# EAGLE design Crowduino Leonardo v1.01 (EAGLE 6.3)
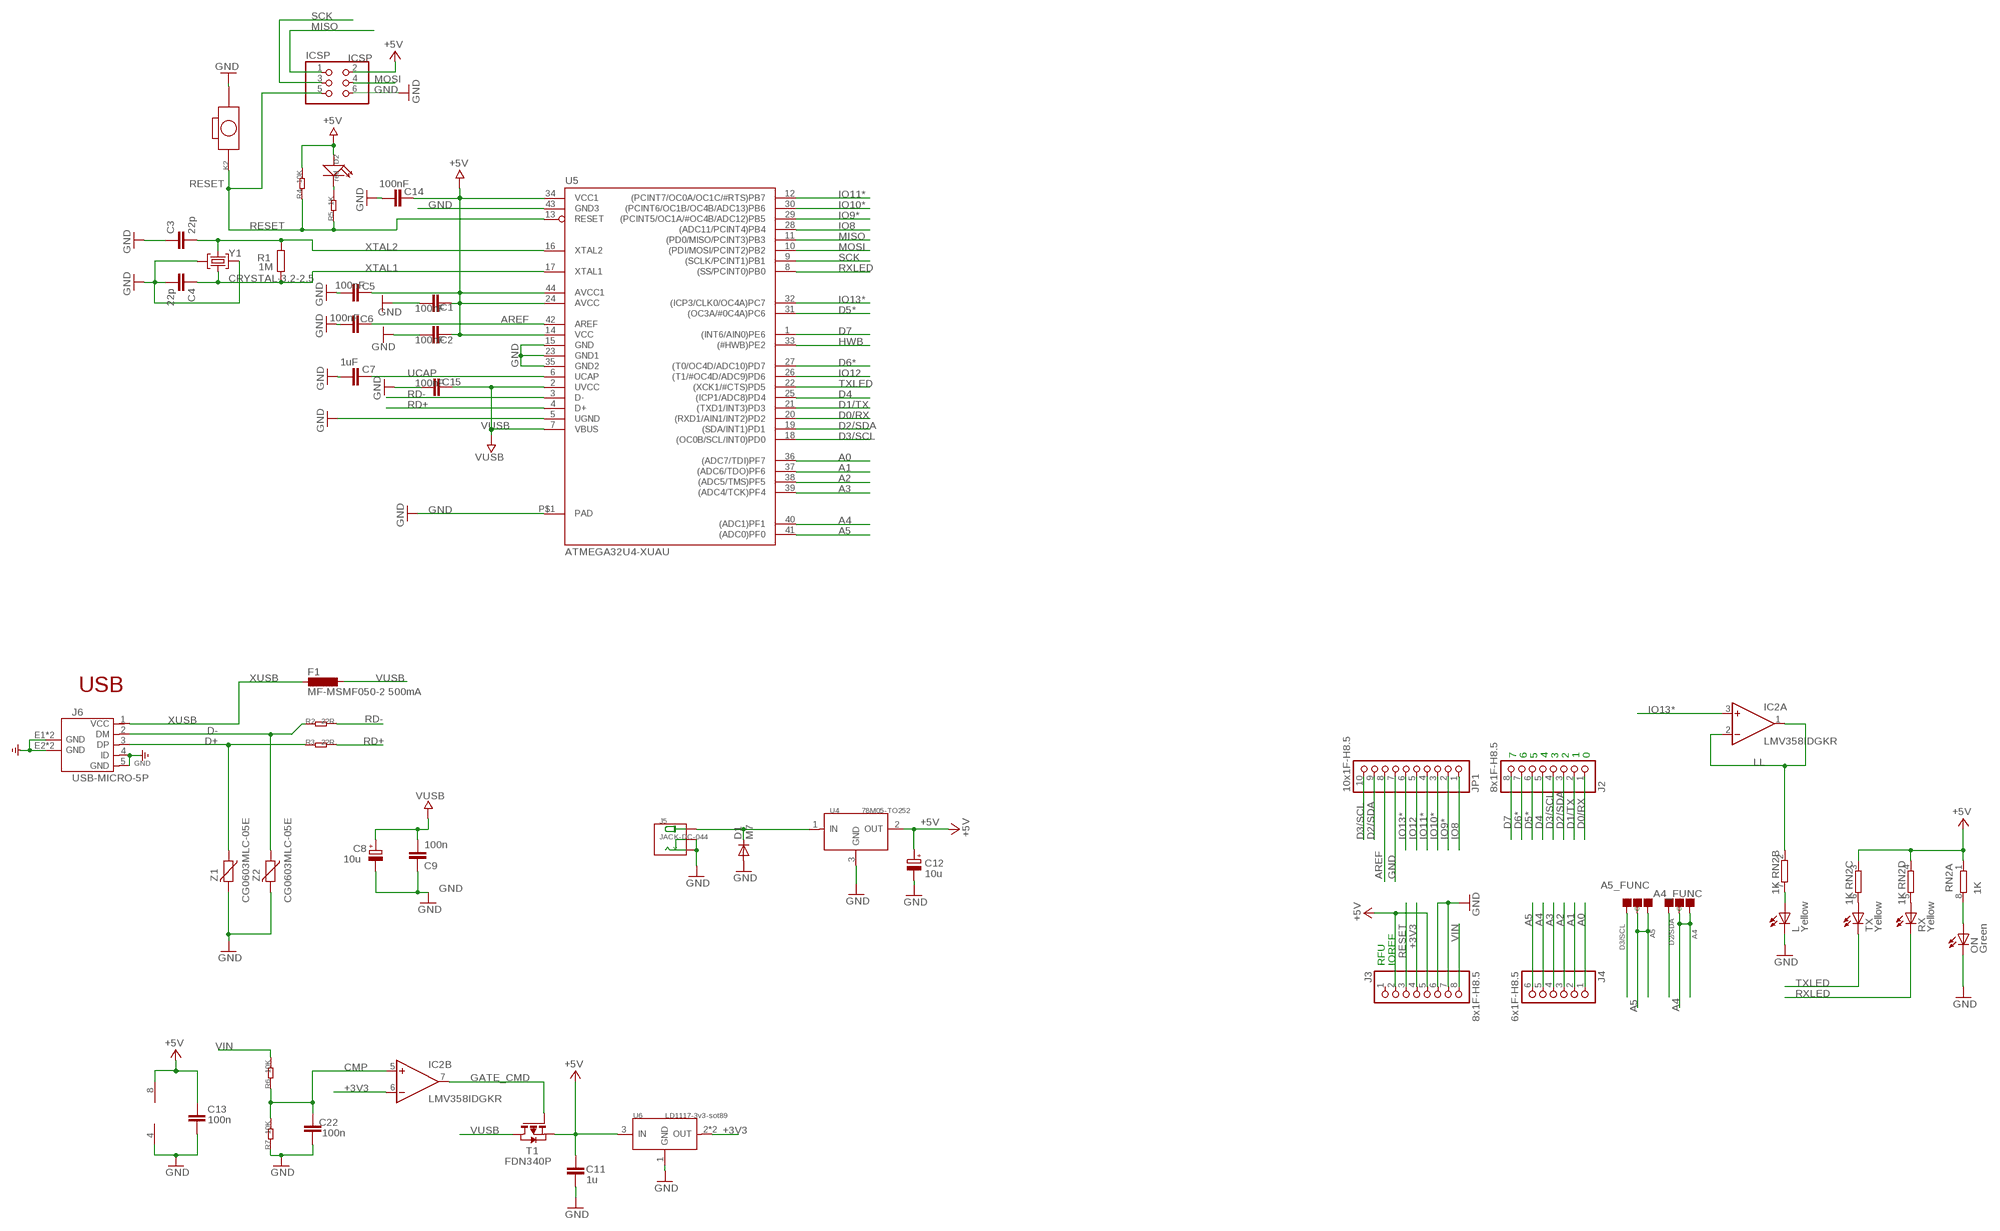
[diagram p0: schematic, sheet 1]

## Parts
A4_FUNC  DNP  PAD-JUMPER-3P-40*40  [3P-SMD-4.1X1.5]
A5_FUNC  DNP  PAD-JUMPER-3P-40*40  [3P-SMD-4.1X1.5]
C1  100nF  C-EUC0603  [C0603-ROUND]
C2  100nF  C-EUC0603  [C0603-ROUND]
C3  22p  C-EUC0603  [C0603-ROUND]
C4  22p  C-EUC0603  [C0603-ROUND]
C5  100nF  C-EUC0603  [C0603-ROUND]
C6  100nF  C-EUC0603  [C0603-ROUND]
C7  1uF  C-EUC0603  [C0603-ROUND]
C8  10u  CPOL-EUSMCB  [SMC_B]
C9  100n  C-EUC0603  [C0603-ROUND]
C11  1u  C-EUC0603  [C0603-ROUND]
C12  10u  CPOL-EUSMCB  [SMC_B]
C13  100n  C-EUC0603  [C0603-ROUND]
C14  100nF  C-EUC0603  [C0603-ROUND]
C15  100nF  C-EUC0603  [C0603-ROUND]
C22  100n  C-EUC0603  [C0603-ROUND]
D1  M7  DIODE-SMB  [SMB]
D2  red  LED'0603'  [LED-0603]
F1  MF-MSMF050-2 500mA  L-EUL1812  [L1812]
IC2  LMV358IDGKR  LMV358MMX  [MSOP08]
ICSP  ICSP  PINHD-2X3  [2X03]
J2  8x1F-H8.5  PINHD-1X8  [1X08]
J3  8x1F-H8.5  PINHD-1X8  [1X08]
J4  6x1F-H8.5  PINHD-1X6  [1X06]
J5  JACK-DC-044  [DC-404]
J6  USB-MICRO-5P  [MICRO-USB-5P]
JP1  10x1F-H8.5  PINHD-1X10  [1X10]
K2  BOTTON-2P-90D  [2P-7.62X3.56-90D]
L  Yellow  LEDCHIPLED_0805  [CHIPLED_0805]
ON  Green  LEDCHIPLED_0805  [CHIPLED_0805]
R1  1M  R-EU_R0603  [R0603-ROUND]
R2  22R  R-0603  [R0603]
R3  22R  R-0603  [R0603]
R4  10K  R-0603  [R0603]
R5  1K  R-0603  [R0603]
R6  10K  R-0603  [R0603]
R7  10K  R-0603  [R0603]
RN2  1K  4R-NCAY16  [CAY16]
RX  Yellow  LEDCHIPLED_0805  [CHIPLED_0805]
T1  FDN340P  PMOSSOT23  [SOT-23]
TX  Yellow  LEDCHIPLED_0805  [CHIPLED_0805]
U4  78M05-TO252  [TO252]
U5  ATMEGA32U4-XUAU  [TQFP44-PAD]
U6  LD1117-3v3-sot89  LD1117'SOT89'  [SOT89]
Y1  CRYSTAL-3.2-2.5  [CRYSTAL-3.2-2.5]
Z1  CG0603MLC-05E  VARISTORCN0603  [CT/CN0603]
Z2  CG0603MLC-05E  VARISTORCN0603  [CT/CN0603]

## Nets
+3V3: IC2.6(B:-IN) J3.4 U6.2(OUT) U6.4(OUT)
+5V [usbvcc]: C1.1 C2.1 C5.1 C11.2 C12.+ C13.1 C14.1 D2.+ IC2.8(P:V+) ICSP.2 J3.2 J3.5 R4.2 RN2.1 RN2.3 RN2.4 T1.2(S) U4.2(OUT) U5.14(VCC) U5.24(AVCC) U5.34(VCC1) U5.44(AVCC1) U6.3(IN)
A0: J4.1 U5.36((ADC7/TDI)PF7)
A1: J4.2 U5.37((ADC6/TDO)PF6)
A2: J4.3 U5.38((ADC5/TMS)PF5)
A3: J4.4 U5.39((ADC4/TCK)PF4)
A4: A4_FUNC.00(L) A4_FUNC.MM(C) J4.5 U5.40((ADC1)PF1)
A5: A5_FUNC.00(L) A5_FUNC.MM(C) J4.6 U5.41((ADC0)PF0)
AREF [aref]: C6.2 JP1.8 U5.42(AREF)
CMP: C22.2 IC2.5(B:+IN) R6.1 R7.2
D0/RX: J2.1 U5.20((RXD1/AIN1/INT2)PD2)
D1/TX: J2.2 U5.21((TXD1/INT3)PD3)
D2/SDA: A4_FUNC.11(R) J2.3 JP1.9 U5.19((SDA/INT1)PD1)
D3/SCL: A5_FUNC.11(R) J2.4 JP1.10 U5.18((OC0B/SCL/INT0)PD0)
D4: J2.5 U5.25((ICP1/ADC8)PD4)
D5*: J2.6 U5.31((OC3A/#0C4A)PC6)
D6*: J2.7 U5.27((T0/OC4D/ADC10)PD7)
D7: J2.8 U5.1((INT6/AIN0)PE6)
D+: J6.3(DP) R3.1 Z1.1
D-: J6.2(DM) R2.1 Z2.1
GATE_CMD: IC2.7(B:OUT) T1.3(G)
GND [gnd]: C1.2 C2.2 C3.1 C4.2 C5.2 C6.1 C7.2 C8.- C9.1 C11.1 C12.- C13.2 C14.2 C15.2 C22.1 D1.A IC2.4(P:V-) ICSP.6 J3.6 J3.7 J5.- J5.CDN J6.4(ID) J6.5(GND) J6.E1(GND) J6.E2(GND) J6.P1(GND) J6.P2(GND) JP1.7 K2.P$2 L.C ON.C R7.1 U4.3(GND) U5.5(UGND) U5.15(GND) U5.23(GND1) U5.35(GND2) U5.43(GND3) U5.P$1(PAD) U6.1(GND) Y1.2(GND) Y1.4(GND) Z1.2 Z2.2
HWB: U5.33((#HWB)PE2)
IO8: JP1.1 U5.28((ADC11/PCINT4)PB4)
IO9*: JP1.2 U5.29((PCINT5/OC1A/#OC4B/ADC12)PB5)
IO10*: JP1.3 U5.30((PCINT6/OC1B/OC4B/ADC13)PB6)
IO11*: JP1.4 U5.12((PCINT7/OC0A/OC1C/#RTS)PB7)
IO12: JP1.5 U5.26((T1/#OC4D/ADC9)PD6)
IO13*: IC2.3(A:+IN) JP1.6 U5.32((ICP3/CLK0/OC4A)PC7)
LL: IC2.1(A:OUT) IC2.2(A:-IN) RN2.2
MISO: ICSP.1 U5.11((PD0/MISO/PCINT3)PB3)
MOSI: ICSP.4 U5.10((PDI/MOSI/PCINT2)PB2)
N$1: D2.- R5.2
N$2: L.A RN2.7
N$3: ON.A RN2.8
N$6: RN2.6 TX.A
N$8: RN2.5 RX.A
RD+: R3.2 U5.4(D+)
RD-: R2.2 U5.3(D-)
RESET: ICSP.5 J3.3 K2.P$1 R4.1 R5.1 U5.13(RESET)
RXLED: RX.C U5.8((SS/PCINT0)PB0)
SCK: ICSP.3 U5.9((SCLK/PCINT1)PB1)
TXLED: TX.C U5.22((XCK1/#CTS)PD5)
UCAP: C7.1 U5.6(UCAP)
VIN [none1]: D1.C J3.8 J5.+ R6.2 U4.1(IN)
VUSB: C8.+ C9.2 C15.1 F1.1 T1.1(D) U5.2(UVCC) U5.7(VBUS)
XTAL1: C4.1 R1.1 U5.17(XTAL1) Y1.1(C1)
XTAL2: C3.2 R1.2 U5.16(XTAL2) Y1.3(C2)
XUSB [usbvcc]: F1.2 J6.1(VCC)
Unconnected: J3.1

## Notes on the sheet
- USB
- 7 | 6 | 5 | 4 | 3 | 2 | 1 | 0
- RFU | IOREF

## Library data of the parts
A4_FUNC A5_FUNC = Discrete:PAD-JUMPER-3P; PARTNO: DNP
C1-C7 C9 C11 C13-C15 C22 = SmartPrj:C-EU: CAPACITOR, European symbol
C8 C12 = rcl:CPOL-EU: POLARIZED CAPACITOR, European symbol
D1 = diode:DIODE-: DIODE
D2 = Discrete:LED*
F1 = rcl:L-EU: INDUCTOR, European symbol
IC2 = linear:LMV358?*: Dual General Purpose, Low Voltage, Rail-to-Rail Output Operational Amplifiers Source: http://www.national.com/mpf/LM/LMV321.html http://www.national.com/dt/lmv_qual.pdf
ICSP = SmartPrj:PINHD-2X3: PIN HEADER
J2 J3 = SmartPrj:PINHD-1X8: PIN HEADER
J4 = SmartPrj:PINHD-1X6: PIN HEADER
J5 = Connector:JACK-DC-044
J6 = Connector:USB-MICRO-5P
JP1 = SmartPrj:PINHD-1X10: PIN HEADER
K2 = Discrete:BOTTON-2P
L ON RX TX = led:LED: LED
R1 = SmartPrj:R-EU_: RESISTOR, European symbol
R2-R7 = Discrete:R*
RN2 = resistor-dil:4R-N: Array Chip Resistor Source: RS Component / Phycomp
T1 = zetex:PMOSSOT23: MOS FET
U4 = IC:78M05: 0.5A Three Terminal Positive Voltage Regulators
U5 = SmartPrj:ATMEGA32U4-XU
U6 = IC:LD1117: Low Drop Fixed And Adjustable Positive Voltage Regulators http://www.datasheetcatalog.org/datasheet/SGSThomsonMicroelectronics/mXuqtqv.pdf
Y1 = SmartPrj:CRYSTAL-3.2-2.5
Z1 Z2 = varistor:VARISTOR: VARISTOR

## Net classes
0 default: width 0.152 mm, drill 0.305 mm, clearance 0.152 mm
2 gnd: width 0.305 mm, drill 0.559 mm, clearance 0.254 mm
3 usbvcc: width 0.254 mm, drill 0.61 mm, clearance 0.254 mm
4 aref: width 0.254 mm, drill 0.61 mm, clearance 0.254 mm

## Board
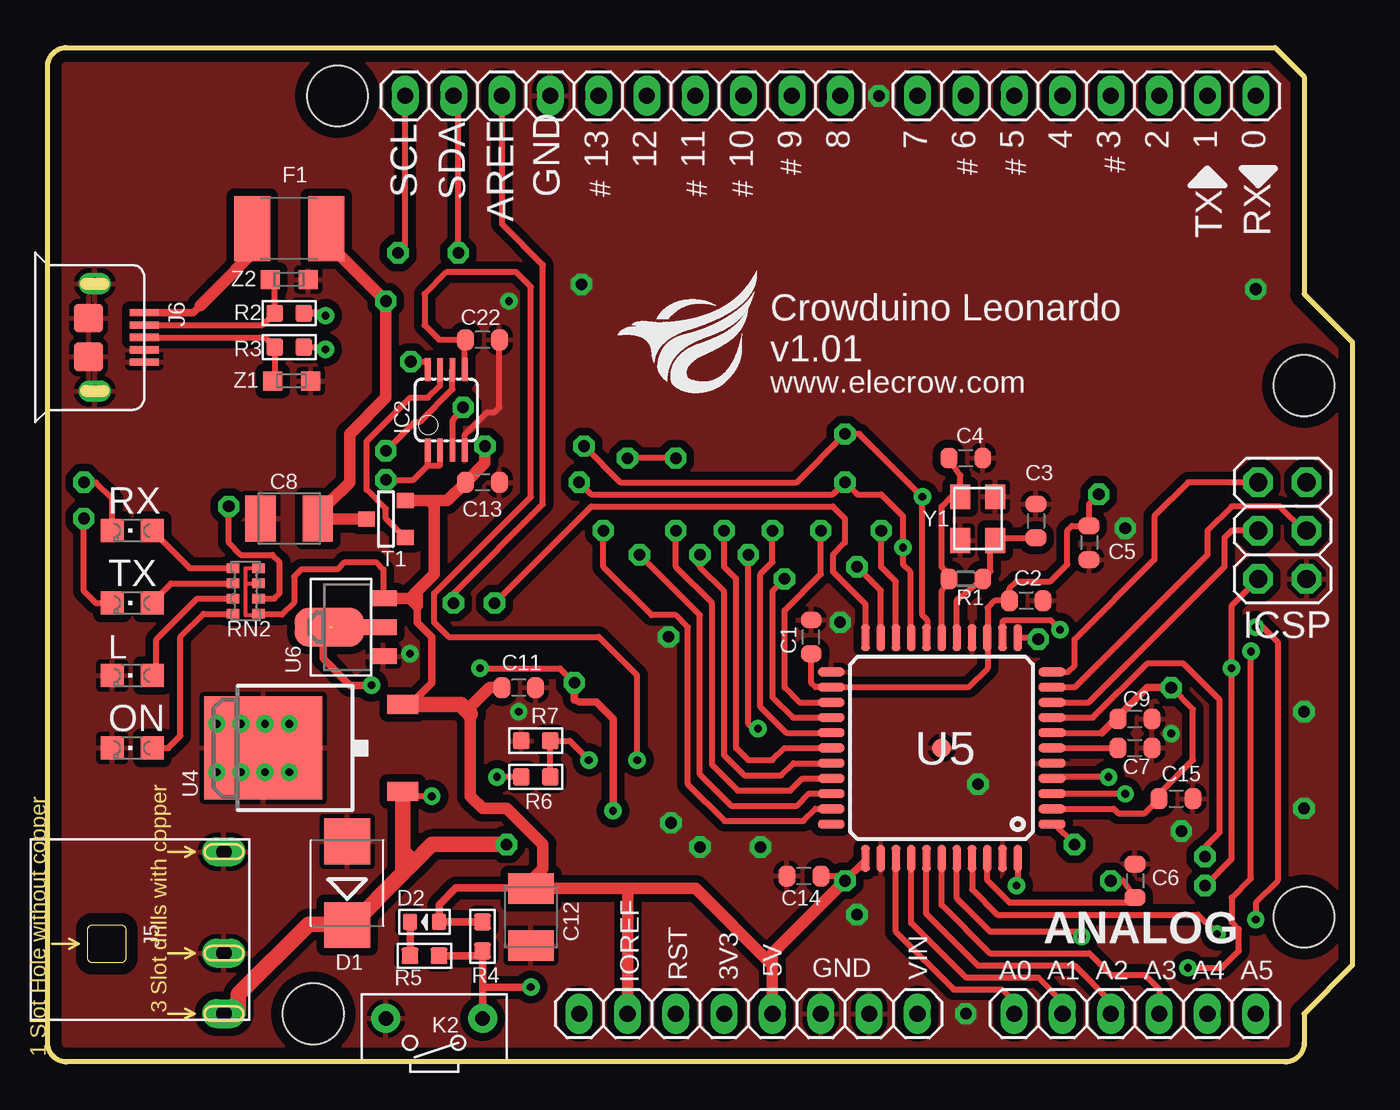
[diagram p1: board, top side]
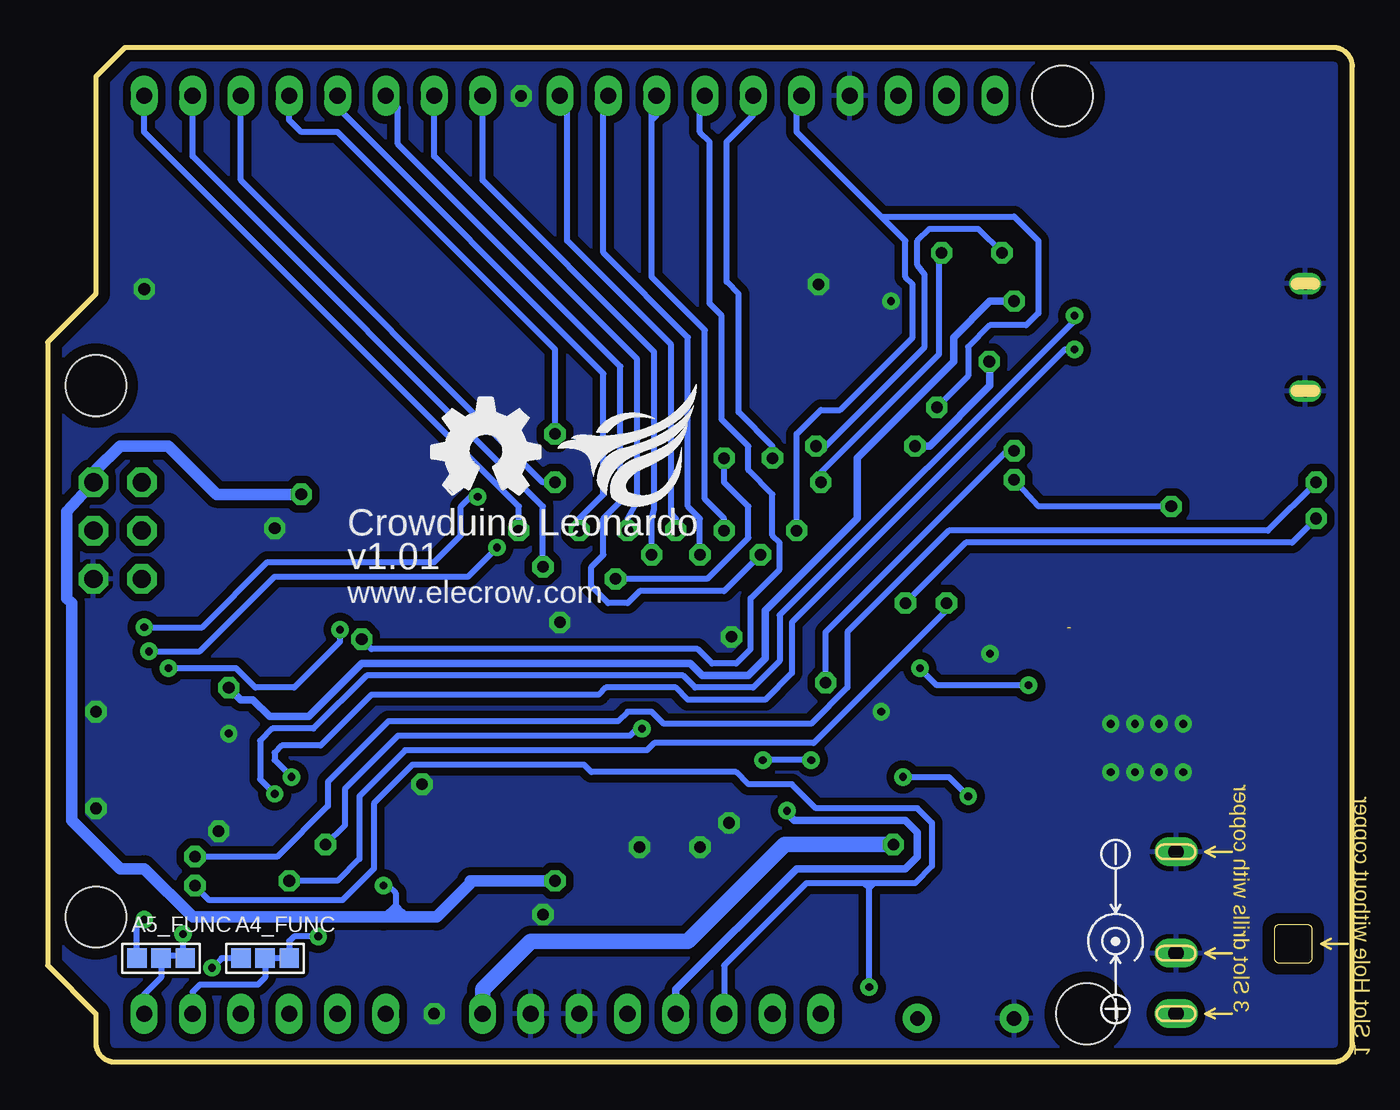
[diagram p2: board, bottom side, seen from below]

Size 68.58 x 53.34 mm. Coordinates in mm from the lower left corner, seen from the top.
Outline: 64.52,53.34 66.04,51.82 66.04,40.39 68.58,37.85 68.58,5.08 66.04,2.54 66.04,1 arc-90 65.04,0 1,0 arc-90 0,1 0,52.34 arc-90 1,53.34 64.52,53.34
Copper layers (1*16): Top 0.035mm / dielectric 1.5mm / Bottom 0.035mm
Design rules "default *": minimum track width 7mil, minimum drill 22mil, track to track 10mil, track to pad 10mil, pad to pad 8mil, via to via 12mil, smd to smd 8mil, copper to edge 24mil, drill to drill 12mil, minimum pad ring 10mil, minimum via ring 10mil, stop-mask expansion 2mil, vias tented up to drill 30mil, thermal gap 10mil
Holes 3.2 mm at 66.04,35.56 66.04,7.62 15.24,50.8 13.97,2.54
vRestrict: area 42.5,38.6 to 43.1,38.9; area 35.8,35.2 to 36.4,35.7; area 44.5,35.2 to 45.2,35.7; area 41.3,35.2 to 41.8,35.7; area 47.9,10.3 to 48.5,10.8; area 50.4,10.2 to 50.9,11

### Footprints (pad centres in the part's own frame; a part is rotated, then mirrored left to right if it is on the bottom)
3P-SMD-4.1X1.5 = smd 1.016 x 1.016: 00 -1.27,0; 11 1.27,0; MM 0,0
C0603-ROUND = smd 0.898 x 1.1: 1 -0.889,0; 2 0.889,0
SMC_B = smd 1.6 x 2.4: + -1.5,0; - 1.5,0
SMB = smd 2.4 x 2.4: A 2.2,0; C -2.2,0
LED-0603 = smd 0.762 x 0.889: + -0.762,0; - 0.762,0
L1812 = smd 1.9 x 3.4: 1 -1.95,0; 2 1.95,0
MSOP08 = smd 0.3 x 1.2: 1 -0.976,-2.113; 2 -0.326,-2.113; 3 0.324,-2.113; 4 0.974,-2.113; 5 0.974,2.112; 6 0.324,2.112; 7 -0.326,2.112; 8 -0.976,2.112
2X03 = drill 0.95 pad 1.55 octagon: 1 -2.54,-1.27; 2 -2.54,1.27; 3 0,-1.27; 4 0,1.27; 5 2.54,-1.27; 6 2.54,1.27
1X08 = drill 0.85 pad 1.422 long: 1 -8.89,0; 2 -6.35,0; 3 -3.81,0; 4 -1.27,0; 5 1.27,0; 6 3.81,0; 7 6.35,0; 8 8.89,0
1X06 = drill 0.85 pad 1.422 long: 1 -6.35,0; 2 -3.81,0; 3 -1.27,0; 4 1.27,0; 5 3.81,0; 6 6.35,0
DC-404 = drill 0.813 pad 1.524 long: + 3.175,10.16; - -5.334,10.16; CDN 0,10.16
MICRO-USB-5P = smd 0.38 x 1.52: 1 -1.3,0; 2 -0.65,0; 3 0,0; 4 0.65,0; 5 1.3,0 | smd 1.524 x 1.524: E1 -1.016,-2.921; E2 1.016,-2.921 | drill 0.635 pad 1.143 long: P1 -2.819,-2.591; P2 2.819,-2.591
1X10 = drill 0.85 pad 1.422 long: 1 -11.43,0; 2 -8.89,0; 3 -6.35,0; 4 -3.81,0; 5 -1.27,0; 6 1.27,0; 7 3.81,0; 8 6.35,0; 9 8.89,0; 10 11.43,0
2P-7.62X3.56-90D = drill 0.762 pad 1.524: P$1 0,2.54; P$2 0,-2.54
CHIPLED_0805 = smd 1.2 x 1.2: A 0,-1.05; C 0,1.05
R0603-ROUND = smd 0.898 x 1.1: 1 -0.889,0; 2 0.889,0
R0603 = smd 0.889 x 0.889: 1 -0.762,0; 2 0.762,0
CAY16 = smd 0.5 x 0.65: 1 -1.2,-0.675; 2 -0.4,-0.675; 3 0.4,-0.675; 4 1.2,-0.675; 5 1.2,0.675; 6 0.4,0.675; 7 -0.4,0.675; 8 -1.2,0.675
SOT-23 = smd 0.787 x 0.889: 1 0.025,-1.016; 2 -0.94,1.016; 3 0.991,1.016
TO252 = smd 1.016 x 1.651: 1 -2.286,-4.826; 2 2.286,-4.826 | smd 5.4 x 6.2: 3 0,2.5
TQFP44-PAD = smd 1.4 x 0.45: 1 -5.8,4; 2 -5.8,3.2; 3 -5.8,2.4; 4 -5.8,1.6; 5 -5.8,0.8; 6 -5.8,0; 7 -5.8,-0.8; 8 -5.8,-1.6; 9 -5.8,-2.4; 10 -5.8,-3.2; 11 -5.8,-4; 23 5.8,-4; 24 5.8,-3.2; 25 5.8,-2.4; 26 5.8,-1.6; 27 5.8,-0.8; 28 5.8,0; 29 5.8,0.8; 30 5.8,1.6; 31 5.8,2.4; 32 5.8,3.2; 33 5.8,4 | smd 0.45 x 1.4: 12 -4,-5.8; 13 -3.2,-5.8; 14 -2.4,-5.8; 15 -1.6,-5.8; 16 -0.8,-5.8; 17 0,-5.8; 18 0.8,-5.8; 19 1.6,-5.8; 20 2.4,-5.8; 21 3.2,-5.8; 22 4,-5.8; 34 4,5.8; 35 3.2,5.8; 36 2.4,5.8; 37 1.6,5.8; 38 0.8,5.8; 39 0,5.8; 40 -0.8,5.8; 41 -1.6,5.8; 42 -2.4,5.8; 43 -3.2,5.8; 44 -4,5.8 | smd 1 x 1: P$1 0,0
SOT89 = smd 0.8 x 1.4: 1 -1.524,-1.905; 3 1.524,-1.905 | smd 0.8 x 1.9: 2 0,-1.651 | smd 2.032 x 3.65: 4 0,0.94
CRYSTAL-3.2-2.5 = smd 1.3 x 1.05: 1 -1.15,-0.925; 2 1.15,-0.925; 3 1.15,0.925; 4 -1.15,0.925
CT/CN0603 = smd 1 x 1: 1 -1,0; 2 1,0

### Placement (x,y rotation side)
A4_FUNC  57.15,5.46 180 bottom
A5_FUNC  62.61,5.46 180 bottom
C1  40.13,22.35 90 top
C2  51.44,24.26 0 top
C3  51.94,28.45 270 top
C4  48.26,31.75 0 top
C5  54.74,27.3 270 top
C6  57.15,9.53 270 top
C7  57.15,16.51 0 top
C8  12.7,28.57 180 top
C9  57.15,18.03 180 top
C11  24.77,19.68 180 top
C12  25.4,7.62 270 top
C13  22.86,30.48 0 top
C14  39.75,9.78 180 top
C15  59.31,13.84 0 top
C22  22.86,37.97 180 top
D1  15.75,9.4 90 top
D2  19.81,7.37 180 top
F1  12.7,43.81 180 top
IC2  20.95,34.29 0 top
ICSP  64.9,27.94 270 top
J2  54.61,50.8 180 top
J3  36.83,2.54 0 top
J4  57.15,2.54 0 top
J5  -0.89,5.71 270 top
J6  5.08,38.1 270 top
JP1  30.23,50.8 180 top
K2  20.32,2.29 270 top
L  4.45,20.32 90 top
ON  4.45,16.51 90 top
R1  48.26,25.4 0 top
R2  12.7,39.37 0 top
R3  12.7,37.59 0 top
R4  22.86,6.6 90 top
R5  19.81,5.59 180 top
R6  25.65,14.99 180 top
R7  25.65,16.89 0 top
RN2  10.41,24.77 90 top
RX  4.45,27.94 90 top
T1  17.78,28.57 270 top
TX  4.45,24.13 90 top
U4  13.84,16.51 90 top
U5  46.99,16.51 180 top
U6  15.75,22.86 90 top
U$1  [ELECROW_NRW_6]  29.97,35.18 0 top
U$2  [ELECROW_NRW_6]  41.78,29.21 0 bottom
U$3  [OSHW_FILLX200_NOTEXT]  48.39,29.84 0 bottom
Y1  48.9,28.57 270 top
Z1  12.83,35.81 0 top
Z2  12.7,41.15 0 top

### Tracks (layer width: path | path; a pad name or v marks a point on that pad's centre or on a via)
+3V3  (via drill 0.41, 0.61)  (1 unrouted)
  Top 0.305: IC2.6 21.28,35.38 19.56,33.66 19.3,33.66 v17.78,32.13 | U6.2 14.99,22.86 14.48,22.35 | v22.73,20.7 26.92,20.7 v27.69,19.94
  Top 0.406: v27.69,19.94 27.69,19.05 27.94,18.92 28.83,18.92 29.72,18.03 v29.72,13.21 | 14.48,22.35 14.48,21.21 15.88,19.81 v17.02,19.81
  Bottom 0.305: v17.78,32.13 17.91,32.13 18.03,32 18.29,32 27.69,22.61 v27.69,19.94 | v17.02,19.81 21.84,19.81 v22.73,20.7
  Bottom 0.406: J3.4 35.56,3.81 29.21,10.16 23.5,10.16 22.86,10.79 22.86,12.06 23.5,12.7 29.34,12.7 29.72,13.08 v29.72,13.21
+5V  (via drill 0.41, 0.61)
  Top 0.203: 10.41,25.16 10.41,23.5 11.02,23.5 RN2.1 | 10.41,25.16 RN2.3 | 10.41,25.16 10.41,25.96 RN2.4
  Top 0.305: IC2.8 19.98,36.83 v19.09,36.83 | RN2.1 11.13,23.53 12.32,23.53 12.95,24.16 12.95,25.53 13.34,25.91 15.24,25.91 15.62,26.29 17.27,26.29 17.65,25.91 U6.3 | C1.1 40.13,19.94 40.36,19.71 U5.24 48.41,19.71 49.4,20.7 49.4,22.32 | 49.4,22.32 49.4,23.88 49.78,24.26 C2.1 50.55,24.89 50.93,25.27 52.7,25.27 53.59,26.16 53.59,27.94 53.85,28.19 C5.1 54.74,29.34 v55.24,29.84 55.63,29.84 | 49.4,22.32 U5.14 | C14.1 41.66,9.78 v41.91,9.53 | U5.44 50.99,9.33 v50.93,9.27
  Top 0.406: 23.46,19.67 C11.2 | v41.91,9.53 42.99,10.61 U5.34 | 25,9.12 C12.+ 25.38,9.14 21.46,9.14 20.57,8.26 D2.+ R4.2 | 18.92,18.8 19.05,18.8 20.19,19.94 20.19,22.35 19.43,23.11 19.43,24
  Top 0.61: 20.07,29.52 20.32,29.26 20.32,25.65 19.43,24.77 | 20.07,29.52 T1.2 | C12.+ 30.48,9.12 | 38.1,5.08 34.06,9.12 30.48,9.12 | 38.1,5.08 J3.5 | 30.48,9.12 J3.2 | 38.1,5.08 38.1,5.71 v41.91,9.53 | 25,9.12 26.04,10.16 26.04,11.43 24.13,13.34 22.86,13.34 22.23,13.97 22.23,18.29 22.23,18.67 23.24,19.68 C11.2 | v22.99,32.38 22.99,31.5 C13.1 21.01,29.52 20.07,29.52 | U6.3 19.05,24.38 | 19.05,24.38 19.43,24.77 | 19.05,24.38 19.43,24 19.43,24.77
  Top 0.813: U4.2 18.92,18.8 21.72,18.8 22.23,18.29
  Bottom 0.305: 50.29,8.26 50.29,8.89 50.67,9.27 v50.93,9.27 | 50.29,8.26 50.93,7.62 | 50.29,8.26 50.29,7.75 | 50.29,8.26 49.91,7.87
  Bottom 0.406: v22.99,32.38 22.23,32.38 19.05,35.56 19.05,36.54 v19.09,36.83
  Bottom 0.61: v55.24,29.84 59.69,29.84 62.23,32.38 64.77,32.38 66.04,31.11 ICSP.2 67.56,28.96 67.56,24.38 67.31,24.13 67.31,12.7 64.77,10.16 63.5,10.16 60.96,7.62 50.93,7.62 48.13,7.62 46.35,9.4 46.35,9.53 v41.91,9.53
A0
  Top 0.305: J4.1 50.8,3.17 50.16,3.81 47.62,3.81 44.59,6.84 U5.36
A1
  Top 0.305: J4.2 53.34,3.17 52.07,4.45 48.26,4.45 45.39,7.32 U5.37
A2
  Top 0.305: J4.3 55.88,3.17 53.98,5.08 48.9,5.08 46.19,7.79 U5.38
A3
  Top 0.305: 58.42,3.17 J4.4 58.42,3.81 57.66,4.57 55.88,4.57 54.74,5.71 49.53,5.71 46.99,8.26 U5.39
A4  (via drill 0.41)
  Top 0.305: U5.40 47.79,8.6 49.53,6.86 54.1,6.86 v54.36,6.6
  Bottom 0.305: J4.5 60.96,3.68 60.58,4.06 57.53,4.06 57.15,4.45 A4_FUNC.MM A4_FUNC.00 55.88,6.35 55.63,6.6 v54.36,6.6
A5  (via drill 0.41)
  Top 0.305: 61.21,6.99 v61.47,6.73 60.45,7.75 49.91,7.75 48.59,9.07 U5.41
  Bottom 0.305: v61.47,6.73 61.47,5.59 | 61.47,5.59 A5_FUNC.00 | 61.47,5.59 62.48,5.59 A5_FUNC.MM 62.61,4.45 63.5,3.56 J4.6
AREF  (via drill 0.61)
  Top 0.305: v21.34,24.13 21.34,24.64 26.04,29.34 26.04,41.91 23.88,44.07 JP1.8 | v55.88,9.53 56.53,9.53 C6.2 56.9,8.38 50.55,8.38 49.39,9.54 U5.42
  Bottom 0.305: v21.34,24.13 21.34,23.75 28.32,16.76 36.7,16.76 37.08,16.38 49.78,16.38 52.2,13.97 52.2,10.67 53.34,9.53 v55.88,9.53
CMP  (via drill 0.41)
  Top 0.305: IC2.5 21.93,37.93 C22.2 20.57,37.97 19.81,38.73 19.81,40.39 20.95,41.53 24.64,41.53 25.4,40.77 25.4,29.72 20.32,24.64 20.32,23.11 21.08,22.35 28.96,22.35 30.99,20.32 v30.99,15.88 | v28.45,15.88 27.43,16.89 R7.2 R6.1
  Bottom 0.305: v28.45,15.88 v30.99,15.88
D0/RX  (via drill 0.61)
  Top 0.305: v43.81,27.94 43.81,26.04 44.59,25.26 U5.20
  Bottom 0.305: v43.81,27.94 43.81,29.21 63.5,48.9 J2.1
D1/TX  (via drill 0.61)
  Top 0.305: v42.55,26.04 43.79,24.79 U5.21
  Bottom 0.305: v42.55,26.04 42.55,29.21 60.96,47.62 J2.2
D2/SDA  (via drill 0.41, 0.61)
  Top 0.305: v27.94,30.48 28.57,29.84 41.27,29.84 v41.91,30.48 42.55,29.84 43.81,29.84 44.96,28.7 v44.96,27.05 44.96,26.16 45.34,25.78 45.34,22.36 U5.19 | JP1.9 21.59,50.55 v21.59,42.55 | v63.25,21.59 63.25,9.65 62.23,8.64 62.23,7.37 62.61,6.99 62.61,5.84 61.72,4.95 v59.94,4.95
  Bottom 0.305: v21.59,42.55 21.59,42.42 21.72,42.29 21.72,37.21 27.94,30.99 v27.94,30.48 | v41.91,30.48 42.55,30.48 58.42,46.35 J2.3 | A4_FUNC.11 59.44,5.46 v59.94,4.95 | v44.96,27.05 46.48,25.53 56.64,25.53 60.58,21.59 v63.25,21.59
D3/SCL  (via drill 0.41, 0.61)
  Top 0.305: v18.41,42.55 18.8,42.93 JP1.10 | v28.19,32.38 30.1,30.48 39.37,30.48 v41.91,33.02 42.67,33.02 v45.97,29.72 45.97,23.5 46.23,23.24 46.23,22.35 U5.18 | v63.5,7.49 63.5,8.38 64.64,9.53 64.64,22.1 63.88,22.86 v63.5,22.86
  Bottom 0.305: v18.41,42.55 19.68,43.81 22.23,43.81 22.86,43.18 22.86,41.91 22.48,41.4 22.48,37.59 27.69,32.38 v28.19,32.38 | v41.91,33.02 41.91,37.47 53.34,48.9 55.24,48.9 55.88,49.53 J2.4 | A5_FUNC.11 63.88,7.11 v63.5,7.49 | v45.97,29.72 46.35,29.72 46.86,29.21 46.86,27.69 48.26,26.29 57.02,26.29 60.45,22.86 v63.5,22.86
D4  (via drill 0.61)
  Top 0.305: v40.64,27.94 40.64,25.65 38.73,23.75 38.73,19.68 39.51,18.91 U5.25
  Bottom 0.305: J2.5 53.34,50.16 39.37,36.2 39.37,29.84 40.64,28.57 v40.64,27.94
D5*  (via drill 0.61)
  Top 0.305: v31.11,26.67 34.29,23.5 34.29,15.11 35.93,13.47 39.38,13.47 40.02,14.11 U5.31
  Bottom 0.305: J2.6 50.16,50.16 50.16,48.26 38.48,36.58 38.48,29.46 39.37,28.57 39.37,26.67 40.01,26.04 40.01,25.02 39.12,24.13 38.1,24.13 37.47,24.77 33.02,24.77 v31.11,26.67
D6*  (via drill 0.61)
  Top 0.305: v38.1,27.94 38.1,26.29 37.47,25.65 37.47,18.67 38.82,17.31 U5.27
  Bottom 0.305: J2.7 48.26,47.62 37.59,36.96 37.59,29.46 38.1,28.57 v38.1,27.94
D7  (via drill 0.41, 0.61)
  Top 0.305: 53.87,11.43 v53.98,11.43 52.9,12.51 U5.1 | v36.83,26.67 36.83,17.78 37.08,17.53 v37.34,17.53
  Bottom 0.305: J2.8 45.72,46.35 36.7,37.34 36.7,29.08 36.83,28.57 v36.83,26.67 | v53.98,11.43 52.96,12.45 52.96,14.35 50.16,17.14 37.97,17.14 37.59,17.53 v37.34,17.53
D+
  Top 0.305: Z1.1 11.94,35.92 R3.1 11.43,38.1 J6.3
D-
  Top 0.305: Z2.1 11.94,40.91 R2.1 11.32,38.75 J6.2
GATE_CMD
  Top 0.305: IC2.7 20.63,35.56 19.99,34.92 19.05,34.92 16.76,32.64 16.76,30.1 17.78,29.08 17.78,28.57 18.77,27.58 T1.3
GND  (via drill 0.41, 0.61)
  Top 0.305: IC2.4 21.93,32.98 23.11,34.16 23.5,34.16 23.75,34.42 C22.1 | v11.43,15.24 v12.7,15.24
  other vias: 37.47,11.3 48.9,14.61 59.59,12.14 41.66,23.11 56.64,28.07 28.07,40.89 34.29,11.3 32.77,12.57 42.55,7.75 66.04,13.34 66.04,18.41 48.26,2.54 43.69,50.8 32.64,22.35 63.5,40.64 19.05,21.46 24.77,18.41 24.26,40.01 59.05,17.27 8.89,17.78 10.16,17.78 11.43,17.78 12.7,17.78 8.89,15.24 10.16,15.24
  pour Bottom (isolate 0.406, rank 2): -1.78,53.72 69.09,53.59 69.09,-0.76 1.51,-0.76 arc-90 -1.65,1.76
  pour Top (isolate 0.406, rank 2): -1.65,53.98 70.99,53.59 71.12,1.64 arc-90 69.61,-0.76 1.13,-0.76 arc-90 -1.52,2.02
IO8  (via drill 0.61)
  Top 0.305: v35.56,27.94 35.56,26.04 36.2,25.4 36.2,16.51 36.83,15.88 38.1,15.88 38.73,16.51 U5.28
  Bottom 0.305: v35.56,27.94 35.56,28.57 35.81,28.83 35.81,37.72 41.27,43.18 41.27,50.42 JP1.1
IO9*  (via drill 0.61)
  Top 0.305: v34.29,26.67 34.29,26.04 35.56,24.77 35.56,16.13 36.61,15.07 38.57,15.07 39.2,15.71 U5.29
  Bottom 0.305: v34.29,26.67 34.29,28.57 34.92,29.21 34.92,38.1 39.37,42.55 39.37,50.55 JP1.2
IO10*  (via drill 0.61)
  Top 0.305: v33.02,27.94 33.02,26.04 34.92,24.13 34.92,15.62 36.27,14.28 39.04,14.28 39.67,14.91 U5.30
  Bottom 0.305: 36.58,50.16 36.58,49.78 36.83,49.53 | 36.58,50.16 JP1.3 | v33.02,27.94 33.02,28.57 34.04,29.59 34.04,38.48 36.83,41.27 36.83,49.91 36.58,50.16
IO11*  (via drill 0.61)
  Top 0.305: 52.16,22.31 v52.07,22.23 51.98,22.31 U5.12
  Bottom 0.305: v52.07,22.23 51.56,21.72 34.42,21.72 33.66,20.95 32.38,20.95 31.62,21.72 31.62,24.38 30.1,25.91 30.1,27.3 30.48,27.69 30.48,29.84 31.75,31.11 31.75,32.38 33.15,33.78 33.15,39.24 33.78,39.88 33.78,48.39 34.29,48.9 34.29,50.55 JP1.4
IO12  (via drill 0.61)
  Top 0.305: v38.73,25.4 38.1,24.77 38.1,19.18 39.17,18.11 U5.26 | v33.02,31.75 v30.48,31.75
  Bottom 0.305: v38.73,25.4 33.91,25.4 31.75,27.56 31.75,29.21 33.02,30.48 v33.02,31.75 | JP1.5 31.5,49.78 32.89,48.39 32.89,41.02 32.26,40.39 32.26,34.16 30.48,32.38 v30.48,31.75
IO13*  (via drill 0.61)
  Top 0.305: v29.21,27.94 29.21,26.04 31.75,23.5 33.02,23.5 33.66,22.86 33.66,14.61 35.59,12.68 39.73,12.68 40.36,13.31 U5.32 | IC2.3 21.28,33.73 v21.84,34.42
  Bottom 0.305: JP1.6 29.21,50.55 29.21,48.9 24.77,44.45 | v21.84,34.42 20.19,36.07 20.19,37.59 19.05,38.73 17.14,38.73 16.51,39.37 16.51,43.18 17.78,44.45 24.77,44.45 | v29.21,27.94 29.21,33.02 27.94,34.29 26.92,34.29 23.11,38.1 23.11,40.89 23.5,41.27 23.5,43.18 24.77,44.45
LL  (via drill 0.61)
  Top 0.305: IC2.2 20.63,31.37 19.98,31.37 | 19.98,31.37 IC2.1 | v17.78,30.61 19.22,30.61 19.98,31.37 | v9.53,29.21 9.53,27.3 10.16,26.67 11.81,26.67 12.19,26.29 12.19,24.64 11.92,24.36 RN2.2
  Bottom 0.305: v17.78,30.61 16.51,29.21 v9.53,29.21
MISO
  Top 0.305: ICSP.1 59.94,30.48 58.17,28.7 58.17,26.42 53.98,22.23 53.98,20.83 53.66,20.51 U5.11
MOSI
  Top 0.305: U5.10 54,19.71 60.96,26.67 60.96,27.94 62.23,29.21 64.77,29.21 66.04,27.94 ICSP.4
N$1
  Top 0.406: D2.- R5.2
N$2
  Top 0.305: RN2.7 7.86,24.36 5.71,22.23 5.71,20.32 L.A
N$3
  Top 0.305: RN2.8 8.2,23.57 6.99,22.35 6.99,17.14 6.35,16.51 ON.A
N$6
  Top 0.305: RN2.6 6.5,25.16 5.5,24.16 TX.A
N$8
  Top 0.305: RN2.5 7.47,25.96 RX.A
RD+  (via drill 0.41)
  Top 0.305: R3.2 14.48,37.59 v14.61,37.47 | v55.75,14.99 52.87,14.99 U5.4
  Bottom 0.305: v14.61,37.47 15.11,37.47 29.46,23.11 29.46,20.45 30.86,19.05 34.92,19.05 35.56,19.68 39.24,19.68 39.62,19.3 51.56,19.3 54.23,16.64 56.26,16.64 56.64,16.26 56.64,15.88 v55.75,14.99
RD-  (via drill 0.41)
  Top 0.305: v56.64,14.1 52.8,14.1 U5.3
  Top 0.406: R2.2 14.48,39.37 v14.61,39.24
  Bottom 0.305: v14.61,39.24 14.61,38.99 30.1,23.5 30.1,21.08 31.5,19.68 34.54,19.68 35.18,20.32 51.82,20.32 54.61,17.53 56.77,17.53 57.4,16.89 57.4,14.86 v56.64,14.1
RESET  (via drill 0.41, 0.61)
  Top 0.305: v60.83,9.27 62.23,10.67 v62.23,20.7 62.23,24 ICSP.5 | U5.13 50.19,23.14 50.29,23.24 52.7,23.24 v53.21,22.73
  Top 0.406: R5.1 22.61,5.59 R4.1 22.86,3.94 | K2.P$1 22.86,3.94 | 22.86,3.94 v25.4,3.94
  Bottom 0.305: J3.3 33.02,5.08 28.7,9.4 25.65,9.4 | v60.83,9.27 60.07,8.51 53.09,8.51 51.44,10.16 51.44,13.59 49.4,15.62 40.39,15.62 40.01,15.24 32.38,15.24 31.75,14.61 29.46,14.61 28.19,13.34 22.86,13.34 22.1,12.57 22.1,10.29 22.99,9.4 25.15,9.4 | 25.15,9.4 25.65,9.4 | v25.4,3.94 25.4,9.14 | 25.4,9.14 25.15,9.4 | 25.4,9.14 25.65,9.4 | v53.21,22.73 53.21,22.1 55.63,19.68 57.66,19.68 58.67,20.7 v62.23,20.7
RXLED  (via drill 0.61)
  Top 0.305: v1.91,30.48 2.54,30.48 3.4,29.62 RX.C | v60.83,10.79 60.83,11.3 61.59,12.06 61.59,19.05 59.69,20.95 57.78,20.95 54.94,18.11 U5.8
  Bottom 0.305: v1.91,30.48 4.45,27.94 21.21,27.94 26.54,22.61 26.54,19.68 28.45,17.78 36.2,17.78 36.83,18.41 38.1,18.41 38.61,17.91 50.67,17.91 53.85,14.73 53.85,13.46 56.52,10.79 v60.83,10.79
SCK
  Top 0.305: U5.9 54.72,18.91 61.85,26.04 61.85,27.56 62.23,27.94 ICSP.3
TXLED  (via drill 0.61)
  Top 0.305: v1.91,28.57 1.91,24.77 2.54,24.13 TX.C | v23.5,24.13 28.57,29.21 41.27,29.21 41.91,28.57 41.91,27.3 41.27,26.67 41.27,25.78 42.99,24.07 U5.22
  Bottom 0.305: v1.91,28.57 3.17,27.3 20.32,27.3 v23.5,24.13
UCAP
  Top 0.305: U5.6 C7.1
VIN  (via drill 0.41, 0.61)
  Top 0.305: v20.19,13.97 18.92,13.97 U4.1 | R6.2 v23.62,14.99
  Top 0.813: v24.13,11.43 20.19,11.43 19.24,10.48 | 19.24,10.48 18.67,9.91 | J5.+ 10.03,2.54 10.03,3.56 13.72,7.24 15.71,7.24 D1.C 15.96,7.2 18.67,9.91 | U4.1 18.67,11.05 | 18.67,11.05 19.24,10.48 | 18.67,11.05 18.67,9.91
  Bottom 0.305: 20.45,14.22 v20.19,13.97 21.21,14.99 v23.62,14.99
  Bottom 0.813: J3.8 45.72,3.81 43.18,6.35 34.92,6.35 29.84,11.43 v24.13,11.43
VUSB  (via drill 0.61)
  Top 0.305: 56.52,17.8 C9.2 | U5.7 55.41,17.31 | U5.2 56.03,13.31 56.26,13.08 57.66,13.08 C15.1 58.42,14.1 60.2,15.88 60.2,18.54 v59.05,19.68
  Top 0.406: 56.52,18.41 56.52,17.8 | 56.52,18.41 57.78,19.68 v59.05,19.68 | 56.52,18.41 55.41,17.31 | 56.52,18.41 C9.2
  Top 0.61: F1.1 15.29,42.5 v17.78,40.01 17.78,34.92 15.88,33.02 15.88,30.48 14.84,29.44 C8.+ 14.86,28.55 T1.1
  Bottom 0.406: v59.05,19.68 58.42,19.05 57.78,19.05 56.9,18.16 54.86,18.16 52.07,20.95 34.8,20.95 34.16,20.32 31.75,20.32 30.86,21.21 30.86,23.75 26.04,28.57 26.04,31.75 20.95,36.83 20.95,38.1 19.05,40.01 v17.78,40.01
XTAL1
  Top 0.305: C4.1 47.97,30.84 Y1.1 47.51,29.73 46.99,29.21 46.99,26.04 47.62,25.4 R1.1 46.99,24.75 U5.17
XTAL2
  Top 0.305: C3.2 49.82,27.56 Y1.3 49.55,27.15 49.55,25.8 R1.2 47.79,24.28 U5.16
XUSB
  Top 0.406: 8.89,40.64 7.65,39.4 J6.1
  Top 0.61: 8.03,39.78 8.89,40.64 10.79,42.55 10.79,43.23 F1.2

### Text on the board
tPlace: 13 | 12 | 11 | 10 | 9 | 8 | 7 | 6 | 5 | 4 | 3 | 2 | 1 | 0 | Crowduino Leonardo | v1.01 | www.elecrow.com
bPlace: Crowduino Leonardo | v1.01 | www.elecrow.com
tNames: # | # | # | # | SCL | SDA | GND | # | # | # | AREF | TX | RX | 5V | ANALOG | GND | IOREF | RST | 3V3 | VIN | A0 | A1 | A2 | A3 | A4 | A5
